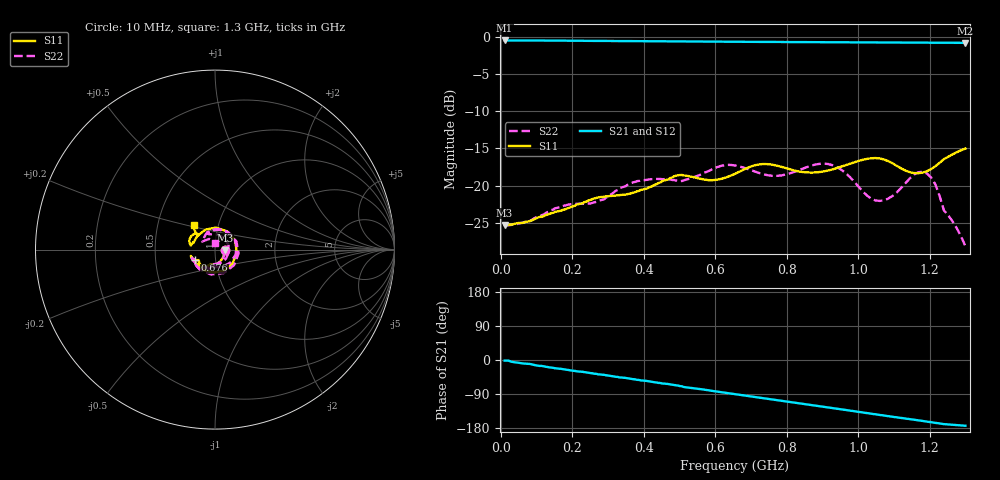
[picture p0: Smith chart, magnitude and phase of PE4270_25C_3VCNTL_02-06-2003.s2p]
!Peregrine Semiconductor Corp.
!S-Parameter Data for Device PE4248 in IL PATH with TEMP = 25C
!File Created On: 02-06-2003
!Start Frequency = 1.000E+01
!Stop Frequency = 1.300E+03
!Number of Points = 145
# MHZ S DB R 75
!Freq  S11MAG  S11PH  S12MAG  S12PH  S21MAG  S21PH  S22MAG  S22PH
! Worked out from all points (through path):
!   145 points, 10 MHz to 1.3 GHz, reference 75 ohm
!   highest |S21| = -0.47 dB at 10 MHz (marker M1); lowest = -0.8 dB at 1.3 GHz (marker M2)
!   group delay of S21, straight-line fit = 377 ps
!   lowest |S11| = -25.3 dB at 10 MHz (marker M3), VSWR 1.11, Z = 83.6 - j0.755 ohm
!   |S11| at or under -10 dB: start of sweep to end of sweep
!   |S22| runs from -28.2 to -17.0 dB; largest |S21 - S12| = 0.53
!   S11 on the Smith chart (normalised r, x): 10 MHz: 1.11, -0.01; 676 MHz: 0.79, -0.09; 1.3 GHz: 0.77, +0.21
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10  -25.32 -4.8  -0.47 -1.7  -0.49 -1.5  -25.33 -4.0
230  -22.37 -74.1  -0.52 -31.3  -0.53 -25.5  -22.46 -72.0
440  -19.68 -117.0  -0.60 -60.3  -0.60 -48.7  -19.12 -110.4
664  -18.21 -151.0  -0.65 -91.4  -0.68 -74.0  -17.39 -144.1
676  -17.94 -152.3  -0.65 -93.0  -0.68 -75.3  -17.55 -146.0
772  -17.32 -161.7  -0.67 -105.8  -0.71 -85.8  -18.70 -149.3
808  -17.80 -93.6  -0.69 -110.6  -0.72 -89.8  -18.37 -151.1
844  -18.18 -7.4  -0.70 -115.6  -0.73 -93.7  -17.74 -156.0
880  -18.24 87.9  -0.71 -120.4  -0.74 -97.5  -17.17 -159.1
904  -18.10 143.2  -0.71 -123.7  -0.74 -100.1  -17.05 -99.4
940  -17.65 164.9  -0.72 -128.6  -0.75 -104.0  -17.51 -9.2
976  -17.08 169.1  -0.73 -133.4  -0.76 -108.0  -18.83 83.2
988  -16.89 167.4  -0.73 -135.0  -0.76 -109.3  -19.44 114.9
1012  -16.55 163.1  -0.73 -138.3  -0.77 -111.9  -20.76 111.6
1060  -16.35 150.8  -0.74 -144.9  -0.78 -117.0  -22.07 -9.6
1096  -17.01 141.4  -0.75 -149.8  -0.79 -120.8  -21.40 -103.0
1120  -17.70 138.0  -0.76 -152.9  -0.80 -123.4  -20.33 -103.2
1156  -18.32 137.6  -0.76 -157.6  -0.81 -127.5  -18.53 -14.6
1192  -18.08 139.4  -0.77 -162.4  -0.82 -131.5  -18.38 65.4
1228  -16.94 138.9  -0.78 -167.4  -0.83 -135.5  -21.44 148.3
1240  -16.44 137.2  -0.78 -169.2  -0.83 -136.7  -23.36 119.2
1300  -15.03 130.4  -0.79 -173.6  -0.85 -140.0  -28.16 88.5
